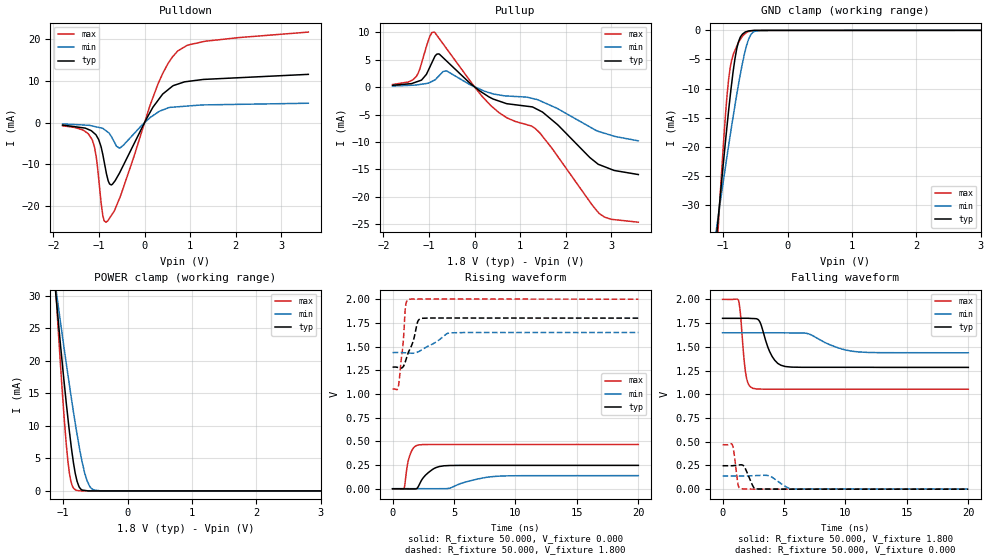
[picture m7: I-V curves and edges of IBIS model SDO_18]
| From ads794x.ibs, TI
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|   SDO 1.8V Model
[Model] SDO_18
Model_type   3-state
Polarity   Non-Inverting
Enable   Active-Low
Vmeas = 0.9
Vref = 0.9
Cref = 15pF
Rref = 50
|   typ   min   max
|   (Nom PVT)   (Fast PVT)  (Slow PVT)
|  (high input impedance)
C_comp   1.7554250e-12   1.4079640e-12   2.1134840e-12
|  (high output)
|C_comp   2.5572700e-12   2.0899950e-12   2.7639340e-12
|  (low output)
|C_comp   1.8338700e-12   1.5069830e-12   2.2101400e-12
[Voltage Range]   1.8   1.65   2
[Temperature Range]   27   125   -40
[Pullup Reference]   1.8   1.65   2
[Pulldown Reference]   0   0   0
[Power Clamp Reference]   1.8   1.65   2
[GND Clamp Reference]   0   0   0
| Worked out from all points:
|   slope of the pulldown table from 0 to 0.27 V, typ, clamps not added: 54.5 ohm
|   slope of the pullup table from 0 to 0.27 V, typ, clamps not added: 171 ohm
|   GND clamp passes 1 mA (typ) near -0.72 V on its own axis
|   POWER clamp passes 1 mA (typ) near -0.77 V on its own axis
|   falling waveform, R_fixture 50.000, V_fixture 1.800: 20-80 % time 876ps typ, 2.16ns min, 379ps max; typ from 1.8 V to 1.28 V
|   rising waveform, R_fixture 50.000, V_fixture 0.000: 20-80 % time 988ps typ, 2.18ns min, 421ps max; typ from 0 V to 0.247 V
|   rising waveform, R_fixture 50.000, V_fixture 1.800: 20-80 % time 769ps typ, 1.57ns min, 372ps max; typ from 1.28 V to 1.8 V
|   falling waveform, R_fixture 50.000, V_fixture 0.000: 20-80 % time 488ps typ, 911ps min, 270ps max; typ from 0.247 V to 0 V
[Pulldown]
|   Voltage   I(typ)   I(min)   I(max)
-1.8V     -610.1uA   -325.1uA   -781uA
-1.352V   -1.269mA   -590.4uA   -1.803mA
-1.152V   -2.131mA   -820.3uA   -4.09mA
-1.058V   -3.112mA   -1.046mA   -8.431mA
-919.3mV  -7.549mA   -1.389mA   -22.15mA
-847.1mV  -11.7mA    -1.969mA   -23.92mA
-732.2mV  -14.96mA   -3.297mA   -22.35mA
-541.2mV  -11.93mA   -6.09mA    -17.99mA
290mV     5.246mA    2.438mA    9.127mA
720.6mV   9.19mA     3.769mA    17.08mA
1.326V    10.36mA    4.232mA    19.5mA
3.595V    11.56mA    4.628mA    21.7mA
[GND Clamp]
|   Voltage   I(typ)   I(min)   I(max)
-1.8V     -125.7mA   -91.16mA   -181.8mA
-1.124V   -38.13mA   -35.79mA   -42.97mA
-1.084V   -33.24mA   -32.64mA   -35.41mA
-1.076V   -32.2mA    -31.98mA   -33.8mA
-963.3mV  -19.03mA   -23.4mA    -14.47mA
-893.8mV  -11.65mA   -18.29mA   -6.632mA
-788.4mV  -3.147mA   -11.02mA   -2.743mA
-734.2mV  -1.197mA   -7.628mA   -1.578mA
-656.7mV  -292.3uA   -3.506mA   -563.1uA
-560.1mV  -51.95uA   -593.2uA   -89.79uA
-394.6mV  -10.96uA   -6.457uA   -32.18uA
3.595V    0A         0A         0A
[Pullup]
|   Voltage   I(typ)   I(min)   I(max)
-1.8V     311.3uA    182.8uA    454uA
-1.287V   902.8uA    358uA      1.835mA
-1.161V   1.298mA    515.7uA    4.437mA
-986.1mV  3.559mA    806.2uA    9.155mA
-887mV    5.307mA    1.225mA    10mA
-786.8mV  6.028mA    1.992mA    8.949mA
-621.1mV  4.791mA    2.953mA    7.065mA
358.5mV   -1.978mA   -1.122mA   -3.386mA
1.254V    -3.601mA   -2.043mA   -7.117mA
1.486V    -4.529mA   -2.675mA   -8.906mA
2.732V    -14.11mA   -8.104mA   -22.99mA
3.595V    -15.93mA   -9.792mA   -24.6mA
[POWER Clamp]
|   Voltage   I(typ)   I(min)   I(max)
-1.8V     111mA      86.6mA     149.7mA
-1.107V   29.49mA    30.69mA    29.66mA
-1.091V   27.75mA    29.49mA    27.04mA
-1.01V    19.23mA    23.66mA    14.74mA
-927.8mV  11.35mA    17.95mA    4.74mA
-875.7mV  6.905mA    14.47mA    1.328mA
-811mV    2.646mA    10.33mA    177.6uA
-748.6mV  566uA      6.656mA    33.53uA
-663mV    74.76uA    2.666mA    6.11uA
-591mV    4.248uA    768.6uA    6.007uA
-523.2mV  4.179uA    145.9uA    5.909uA
3.595V    0A         0A         0A
[Ramp]
R_load = 50
|   typ   min   max
dV/dt_r   0.148095/9.83382e-010 0.0815333/2.16343e-009  0.280328/4.20434e-010
dV/dt_f   0.309993/8.68754e-010  0.128231/2.14486e-009  0.568043/3.7849e-010
[Falling Waveform]
R_fixture = 50.000
V_fixture = 1.800
V_fixture_min = 1.650
V_fixture_max = 2.000
C_fixture = 0.000
|  time   V(typ)   V(min)   V(max)
0s        1.8V       1.648V     2V
1.299ns   1.8V       1.648V     1.989V
1.448ns   1.8V       1.648V     1.858V
1.895ns   1.801V     1.648V     1.211V
2.475ns   1.798V     1.648V     1.062V
3.027ns   1.764V     1.648V     1.055V
4.055ns   1.394V     1.648V     1.053V
5.119ns   1.292V     1.647V     1.053V
10.56ns   1.284V     1.453V     1.053V
20ns      1.283V     1.437V     1.053V
[Rising Waveform]
R_fixture = 50.000
V_fixture = 0.000
V_fixture_min = 0.000
V_fixture_max = 0.000
C_fixture = 0.000
|  time   V(typ)   V(min)   V(max)
0s        16.75uV    1.935mV    -1.243uV
922.8ps   -778.8uV   1.557mV    219.2uV
1.205ns   -1.724mV   1.442mV    250mV
1.397ns   -2.088mV   1.363mV    349.5mV
1.721ns   -1.973mV   1.23mV     434mV
2.131ns   32.86mV    1.063mV    462.5mV
2.929ns   172.7mV    735.7uV    466.9mV
4.173ns   242.2mV    928.5uV    467.1mV
8.641ns   246.7mV    133.2mV    467.2mV
20ns      246.8mV    138.6mV    467.2mV
[Rising Waveform]
R_fixture = 50.000
V_fixture = 1.800
V_fixture_min = 1.650
V_fixture_max = 2.000
C_fixture = 0.000
|  time   V(typ)   V(min)   V(max)
0s        1.283V     1.437V     1.053V
490.3ps   1.279V     1.438V     1.093V
858.5ps   1.288V     1.436V     1.536V
1.048ns   1.343V     1.434V     1.916V
1.303ns   1.445V     1.432V     1.998V
1.67ns    1.553V     1.43V      2.001V
2.041ns   1.762V     1.442V     2.001V
2.355ns   1.798V     1.464V     2.001V
4.725ns   1.801V     1.645V     2.001V
20ns      1.8V       1.648V     2V
[Falling Waveform]
R_fixture = 50.000
V_fixture = 0.000
V_fixture_min = 0.000
V_fixture_max = 0.000
C_fixture = 0.000
|  time   V(typ)   V(min)   V(max)
0s        246.8mV    138.6mV    467.2mV
804.5ps   246.7mV    138.6mV    464.8mV
928.9ps   248.6mV    138.6mV    383.7mV
1.264ns   253.6mV    138.6mV    47.37mV
1.523ns   256.4mV    138.6mV    4.481mV
1.791ns   231.5mV    138.6mV    1.983mV
2.754ns   2.28mV     143.3mV    88.6uV
3.765ns   1.341mV    141.4mV    73.33uV
5.726ns   75.12uV    1.895mV    64.33uV
20ns      16.75uV    1.935mV    -1.243uV
